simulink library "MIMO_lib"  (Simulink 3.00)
libraries: MIMO_lib x68, simulink3 x1

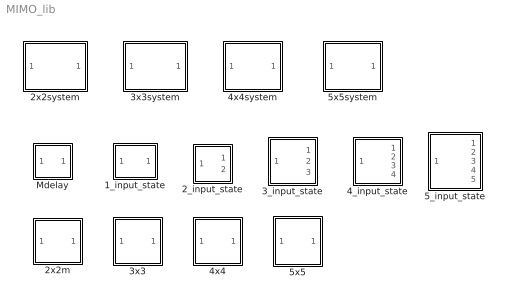
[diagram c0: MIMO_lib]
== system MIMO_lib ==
  1_input_state : Subsystem  mask(SISO_MSF){Ds=}
      mask prompts: Ds "D(s) :"
      mask help: The SISO_MSF block produce, from the input u, a state vector of signal [ ... x''', x'' , x' , x ] to be used further by the K(s) block.
  2_input_state : Subsystem  mask(2_input_state){Ds=}
      mask prompts: Ds "D(s) :"
      mask help: The block generate the state vectors of signal [ ..., x''', x'', x' , x ] of each 2 input signals.
  2x2m : Subsystem  mask(diagonal transferfunction matrix){num=, den=}
      mask prompts: num "diagonal cell array of numurator polynomial"; den "diagonal cell array of denominator polynomial"
      mask help: A block for the simulation of diagonal transfer function matrix, for example the prefilter, and qd part of the feed back controller.
  2x2system : Subsystem  mask(2x2 system){num=, den=, dead=}
      mask prompts: num "numerator :"; den "denominator:"; dead "dead time:"
      mask help: The system is described by a cell array of numerator polynomial, a cell array denominator polynomial of s , and a cell array of dead time.
  3_input_state : Subsystem  mask(3_input_state){Ds=}
      mask prompts: Ds "D(s) :"
      mask help: The block generate the state vectors of signal [ ..., x''', x'', x' , x ] of each 3 input signals.
  3x3 : Subsystem  mask(diagonal transfer function matrix){num=, den=}
      mask prompts: num "diagonal cell array of numurator polynomial"; den "diagonal cell array of denominator polynomial"
      mask help: A block for the simulation of diagonal transfer function matrix, for example the prefilter, and qd part of the feed back controller.
  3x3system : Subsystem  mask(3x3 system){num=, den=, dead=}
      mask prompts: num "numerator"; den "denominator :"; dead "dead time :"
      mask help: The system is described by a cell array of numerator polynomial, a cell array denominator polynomial of s , and a cell array of dead time.
  4_input_state : Subsystem  mask(4_input_state){Ds=}
      mask prompts: Ds "D(s) :"
      mask help: The block generate the state vectors of signal [ ..., x''', x'', x' , x ] of each 4 input signals.
  4x4 : Subsystem  mask(diagonal transfer function matrix){num=, den=}
      mask prompts: num "diagonal cell array of numurator polynomial"; den "diagonal cell array of denominator polynomial"
      mask help: A block for the simulation of diagonal transfer function matrix, for example the prefilter, and qd part of the feed back controller.
  4x4system : Subsystem  mask(4x4 system){num=, den=, dead=}
      mask prompts: num "numerator :"; den "denominator :"; dead "dead time :"
      mask help: The system is described by a cell array of numerator polynomial, a cell array denominator polynomial of s , and a cell array of dead time.
  5_input_state : Subsystem  mask(5_input_state){Ds=}
      mask prompts: Ds "D(s) :"
      mask help: The block generate the state vectors of signal [ ..., x''', x'', x' , x ] of each 5 input signals.
  5x5 : Subsystem  mask(diagonal transfer function matrix){num=, den=}
      mask prompts: num "diagonal cell array of numurator polynomial"; den "diagonal cell array of denominator polynomial"
      mask help: A block for the simulation of diagonal transfer function matrix, for example the prefilter, and qd part of the feed back controller.
  5x5system : Subsystem  mask(5x5 system){num=, den=, dead=}
      mask prompts: num "numerator :"; den "denominator :"; dead "dead time :"
      mask help: The system is described by a cell array of numerator polynomial, a cell array denominator polynomial of s , and a cell array of dead time.
  Mdelay : Subsystem  mask(Mdelay){Mdelay=}
      mask prompts: Mdelay "Delay time:"
      mask help: The modified transport delay that directly feed the signal through when delay time = 0 (to avoid warning if the original Transport delay block is used)

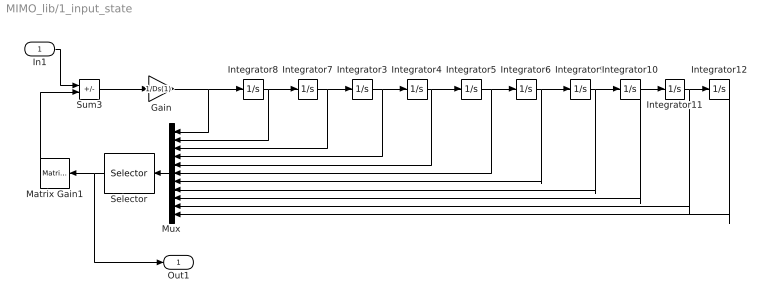
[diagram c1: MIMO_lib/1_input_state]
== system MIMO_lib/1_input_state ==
  In1 : Inport  Port=1  PortWidth=-1  SampleTime=-1  DataType=auto
  Gain : Gain  Gain=1/Ds(1)  SaturateOnIntegerOverflow=on
  Integrator{3..12} (10 alike) : Integrator  ExternalReset=none  InitialConditionSource=internal  InitialCondition=0  LimitOutput=off  UpperSaturationLimit=inf  LowerSaturationLimit=-inf  ShowSaturationPort=off  ShowStatePort=off  AbsoluteTolerance=auto
  Matrix Gain1 : simulink3/Math/Matrix Gain  Orientation=left  K=[0 Ds(2:end)]
  Mux : Mux  Orientation=left  Inputs=11
  Selector : Selector  Orientation=left  Elements=[1 :length(Ds)]  InputPortWidth=11
  Sum3 : Sum  Inputs=+-  SaturateOnIntegerOverflow=on
  Out1 : Outport  Port=1
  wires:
  Sum3/1 -> Gain/1
  In1/1 -> Sum3/1
  Matrix Gain1/1 -> Sum3/2
  Gain/1 -> Integrator8/1, Mux/1
  Integrator8/1 -> Integrator7/1, Mux/2
  Integrator7/1 -> Integrator3/1, Mux/3
  Integrator3/1 -> Integrator4/1, Mux/4
  Integrator4/1 -> Integrator5/1, Mux/5
  Integrator5/1 -> Integrator6/1, Mux/6
  Integrator6/1 -> Integrator9/1, Mux/7
  Integrator9/1 -> Integrator10/1, Mux/8
  Integrator10/1 -> Integrator11/1, Mux/9
  Integrator11/1 -> Integrator12/1, Mux/10
  Integrator12/1 -> Mux/11
  Mux/1 -> Selector/1
  Selector/1 -> Matrix Gain1/1, Out1/1

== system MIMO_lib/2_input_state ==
  In1 : Inport  Port=1  PortWidth=-1  SampleTime=-1  DataType=auto
  1_input_state : MIMO_lib/1_input_state  Ds=Ds{1}
  1_input_state1 : MIMO_lib/1_input_state  Ds=Ds{2}
  Demux : Demux  Outputs=2
  Out1 : Outport  Port=1
  Out2 : Outport  Port=2
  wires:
  Demux/1 -> 1_input_state/1
  Demux/2 -> 1_input_state1/1
  1_input_state/1 -> Out1/1
  In1/1 -> Demux/1
  1_input_state1/1 -> Out2/1

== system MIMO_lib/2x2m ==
  In1 : Inport  Port=1  PortWidth=-1  SampleTime=-1  DataType=auto
  Demux : Demux  Outputs=2
  Mux : Mux  Inputs=2
  Transfer Fcn : TransferFcn  Numerator=num{1,1}  Denominator=den{1,1}
  Transfer Fcn1 : TransferFcn  Numerator=num{2,2}  Denominator=den{2,2}
  Out1 : Outport  Port=1
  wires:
  Demux/1 -> Transfer Fcn/1
  Demux/2 -> Transfer Fcn1/1
  Transfer Fcn/1 -> Mux/1
  Transfer Fcn1/1 -> Mux/2
  Mux/1 -> Out1/1
  In1/1 -> Demux/1

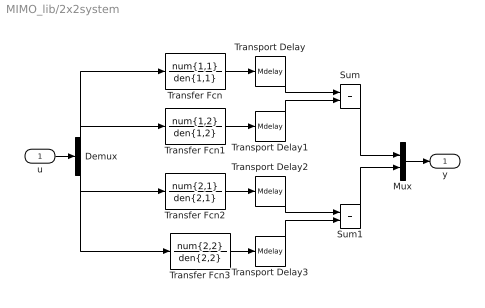
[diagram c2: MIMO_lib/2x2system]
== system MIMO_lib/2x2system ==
  u : Inport  Port=1  PortWidth=-1  SampleTime=-1  DataType=auto
  Demux : Demux  Outputs=2
  Mux : Mux  Inputs=2
  Sum : Sum  Inputs=|++  SaturateOnIntegerOverflow=on
  Sum1 : Sum  Inputs=|++  SaturateOnIntegerOverflow=on
  Transfer Fcn : TransferFcn  Numerator=num{1,1}  Denominator=den{1,1}
  Transfer Fcn1 : TransferFcn  Numerator=num{1,2}  Denominator=den{1,2}
  Transfer Fcn2 : TransferFcn  Numerator=num{2,1}  Denominator=den{2,1}
  Transfer Fcn3 : TransferFcn  Numerator=num{2,2}  Denominator=den{2,2}
  Transport Delay : MIMO_lib/Mdelay  Mdelay=dead{1,1}
  Transport Delay1 : MIMO_lib/Mdelay  Mdelay=dead{1,2}
  Transport Delay2 : MIMO_lib/Mdelay  Mdelay=dead{2,1}
  Transport Delay3 : MIMO_lib/Mdelay  Mdelay=dead{2,2}
  y : Outport  Port=1
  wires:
  Transfer Fcn/1 -> Transport Delay/1
  Transfer Fcn1/1 -> Transport Delay1/1
  Transport Delay/1 -> Sum/1
  Transport Delay1/1 -> Sum/2
  Demux/1 -> Transfer Fcn/1, Transfer Fcn2/1
  Demux/2 -> Transfer Fcn1/1, Transfer Fcn3/1
  Transfer Fcn2/1 -> Transport Delay2/1
  Transfer Fcn3/1 -> Transport Delay3/1
  Transport Delay2/1 -> Sum1/1
  Transport Delay3/1 -> Sum1/2
  Sum/1 -> Mux/1
  Sum1/1 -> Mux/2
  u/1 -> Demux/1
  Mux/1 -> y/1

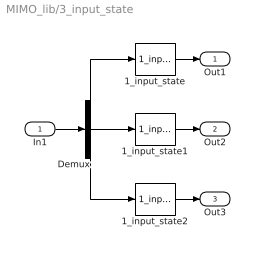
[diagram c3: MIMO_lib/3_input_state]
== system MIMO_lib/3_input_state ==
  In1 : Inport  Port=1  PortWidth=-1  SampleTime=-1  DataType=auto
  1_input_state : MIMO_lib/1_input_state  Ds=Ds{1}
  1_input_state1 : MIMO_lib/1_input_state  Ds=Ds{2}
  1_input_state2 : MIMO_lib/1_input_state  Ds=Ds{3}
  Demux : Demux  Outputs=3
  Out1 : Outport  Port=1
  Out2 : Outport  Port=2
  Out3 : Outport  Port=3
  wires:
  Demux/1 -> 1_input_state/1
  Demux/2 -> 1_input_state1/1
  1_input_state/1 -> Out1/1
  In1/1 -> Demux/1
  1_input_state1/1 -> Out2/1
  1_input_state2/1 -> Out3/1
  Demux/3 -> 1_input_state2/1

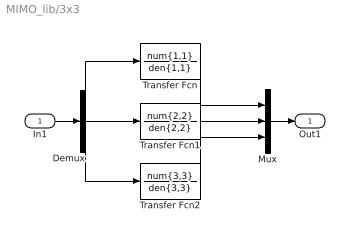
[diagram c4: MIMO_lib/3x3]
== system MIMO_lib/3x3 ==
  In1 : Inport  Port=1  PortWidth=-1  SampleTime=-1  DataType=auto
  Demux : Demux  Outputs=3
  Mux : Mux  Inputs=3
  Transfer Fcn : TransferFcn  Numerator=num{1,1}  Denominator=den{1,1}
  Transfer Fcn1 : TransferFcn  Numerator=num{2,2}  Denominator=den{2,2}
  Transfer Fcn2 : TransferFcn  Numerator=num{3,3}  Denominator=den{3,3}
  Out1 : Outport  Port=1
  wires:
  Transfer Fcn/1 -> Mux/1
  Transfer Fcn1/1 -> Mux/2
  Transfer Fcn2/1 -> Mux/3
  Demux/2 -> Transfer Fcn1/1
  Demux/1 -> Transfer Fcn/1
  Demux/3 -> Transfer Fcn2/1
  Mux/1 -> Out1/1
  In1/1 -> Demux/1

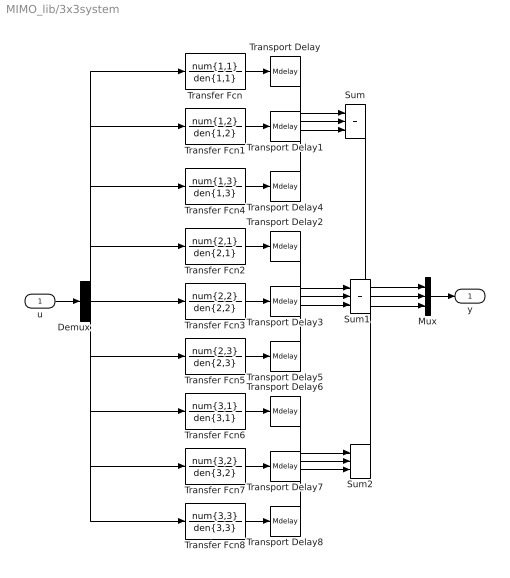
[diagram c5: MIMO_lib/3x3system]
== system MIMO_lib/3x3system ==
  u : Inport  Port=1  PortWidth=-1  SampleTime=-1  DataType=auto
  Demux : Demux  Outputs=3
  Mux : Mux  Inputs=3
  Sum : Sum  Inputs=|+++  SaturateOnIntegerOverflow=on
  Sum1 : Sum  Inputs=|+++  SaturateOnIntegerOverflow=on
  Sum2 : Sum  Inputs=|+++  SaturateOnIntegerOverflow=on
  Transfer Fcn : TransferFcn  Numerator=num{1,1}  Denominator=den{1,1}
  Transfer Fcn1 : TransferFcn  Numerator=num{1,2}  Denominator=den{1,2}
  Transfer Fcn2 : TransferFcn  Numerator=num{2,1}  Denominator=den{2,1}
  Transfer Fcn3 : TransferFcn  Numerator=num{2,2}  Denominator=den{2,2}
  Transfer Fcn4 : TransferFcn  Numerator=num{1,3}  Denominator=den{1,3}
  Transfer Fcn5 : TransferFcn  Numerator=num{2,3}  Denominator=den{2,3}
  Transfer Fcn6 : TransferFcn  Numerator=num{3,1}  Denominator=den{3,1}
  Transfer Fcn7 : TransferFcn  Numerator=num{3,2}  Denominator=den{3,2}
  Transfer Fcn8 : TransferFcn  Numerator=num{3,3}  Denominator=den{3,3}
  Transport Delay : MIMO_lib/Mdelay  Mdelay=dead{1,1}
  Transport Delay1 : MIMO_lib/Mdelay  Mdelay=dead{1,2}
  Transport Delay2 : MIMO_lib/Mdelay  Mdelay=dead{2,1}
  Transport Delay3 : MIMO_lib/Mdelay  Mdelay=dead{2,2}
  Transport Delay4 : MIMO_lib/Mdelay  Mdelay=dead{1,3}
  Transport Delay5 : MIMO_lib/Mdelay  Mdelay=dead{2,3}
  Transport Delay6 : MIMO_lib/Mdelay  Mdelay=dead{3,1}
  Transport Delay7 : MIMO_lib/Mdelay  Mdelay=dead{3,2}
  Transport Delay8 : MIMO_lib/Mdelay  Mdelay=dead{3,3}
  y : Outport  Port=1
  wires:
  Transfer Fcn/1 -> Transport Delay/1
  Transfer Fcn1/1 -> Transport Delay1/1
  Sum/1 -> Mux/1
  Sum1/1 -> Mux/2
  Transfer Fcn2/1 -> Transport Delay2/1
  Transport Delay/1 -> Sum/1
  Transport Delay1/1 -> Sum/2
  Transfer Fcn4/1 -> Transport Delay4/1
  Transfer Fcn3/1 -> Transport Delay3/1
  Transfer Fcn5/1 -> Transport Delay5/1
  Transport Delay2/1 -> Sum1/1
  Demux/1 -> Transfer Fcn/1, Transfer Fcn2/1, Transfer Fcn6/1
  Demux/2 -> Transfer Fcn1/1, Transfer Fcn3/1, Transfer Fcn7/1
  Demux/3 -> Transfer Fcn4/1, Transfer Fcn5/1, Transfer Fcn8/1
  Transport Delay3/1 -> Sum1/2
  Transport Delay5/1 -> Sum1/3
  Transfer Fcn6/1 -> Transport Delay6/1
  Transfer Fcn7/1 -> Transport Delay7/1
  Transfer Fcn8/1 -> Transport Delay8/1
  Transport Delay6/1 -> Sum2/1
  Transport Delay7/1 -> Sum2/2
  Transport Delay8/1 -> Sum2/3
  Sum2/1 -> Mux/3
  Mux/1 -> y/1
  u/1 -> Demux/1
  Transport Delay4/1 -> Sum/3

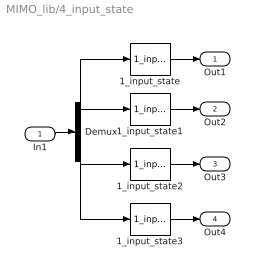
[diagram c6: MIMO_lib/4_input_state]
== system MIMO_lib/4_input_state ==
  In1 : Inport  Port=1  PortWidth=-1  SampleTime=-1  DataType=auto
  1_input_state : MIMO_lib/1_input_state  Ds=Ds{1}
  1_input_state1 : MIMO_lib/1_input_state  Ds=Ds{2}
  1_input_state2 : MIMO_lib/1_input_state  Ds=Ds{3}
  1_input_state3 : MIMO_lib/1_input_state  Ds=Ds{4}
  Demux : Demux  Outputs=4
  Out1 : Outport  Port=1
  Out2 : Outport  Port=2
  Out3 : Outport  Port=3
  Out4 : Outport  Port=4
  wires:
  Demux/1 -> 1_input_state/1
  1_input_state/1 -> Out1/1
  In1/1 -> Demux/1
  1_input_state1/1 -> Out2/1
  1_input_state2/1 -> Out3/1
  Demux/3 -> 1_input_state2/1
  1_input_state3/1 -> Out4/1
  Demux/2 -> 1_input_state1/1
  Demux/4 -> 1_input_state3/1

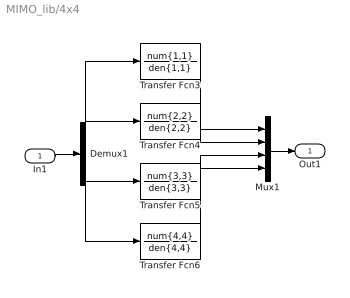
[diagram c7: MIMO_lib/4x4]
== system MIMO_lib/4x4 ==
  In1 : Inport  Port=1  PortWidth=-1  SampleTime=-1  DataType=auto
  Demux1 : Demux  Outputs=4
  Mux1 : Mux  Inputs=4
  Transfer Fcn3 : TransferFcn  Numerator=num{1,1}  Denominator=den{1,1}
  Transfer Fcn4 : TransferFcn  Numerator=num{2,2}  Denominator=den{2,2}
  Transfer Fcn5 : TransferFcn  Numerator=num{3,3}  Denominator=den{3,3}
  Transfer Fcn6 : TransferFcn  Numerator=num{4,4}  Denominator=den{4,4}
  Out1 : Outport  Port=1
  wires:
  Transfer Fcn3/1 -> Mux1/1
  Transfer Fcn5/1 -> Mux1/3
  Demux1/1 -> Transfer Fcn3/1
  Demux1/3 -> Transfer Fcn5/1
  Demux1/4 -> Transfer Fcn6/1
  Transfer Fcn4/1 -> Mux1/2
  Demux1/2 -> Transfer Fcn4/1
  Transfer Fcn6/1 -> Mux1/4
  Mux1/1 -> Out1/1
  In1/1 -> Demux1/1

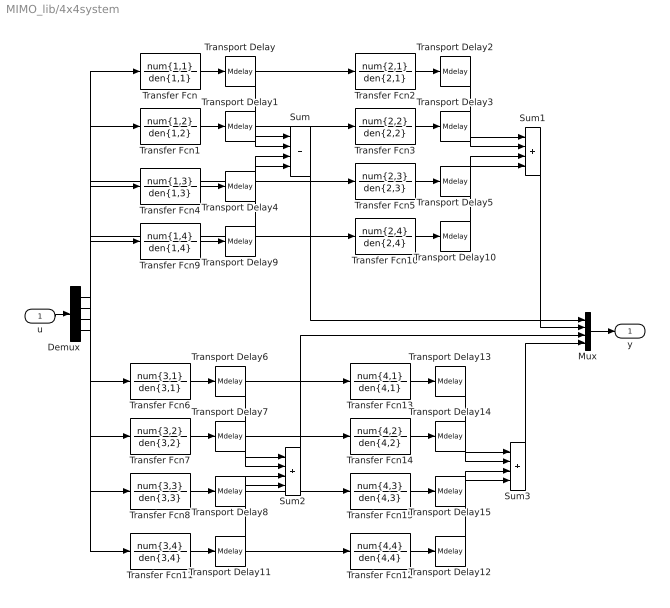
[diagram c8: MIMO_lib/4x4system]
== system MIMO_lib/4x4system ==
  u : Inport  Port=1  PortWidth=-1  SampleTime=-1  DataType=auto
  Demux : Demux  Outputs=4
  Mux : Mux  Inputs=4
  Sum{,1..3} (4 alike) : Sum  Inputs=|++++  SaturateOnIntegerOverflow=on
  Transfer Fcn : TransferFcn  Numerator=num{1,1}  Denominator=den{1,1}
  Transfer Fcn1 : TransferFcn  Numerator=num{1,2}  Denominator=den{1,2}
  Transfer Fcn10 : TransferFcn  Numerator=num{2,4}  Denominator=den{2,4}
  Transfer Fcn11 : TransferFcn  Numerator=num{3,4}  Denominator=den{3,4}
  Transfer Fcn12 : TransferFcn  Numerator=num{4,4}  Denominator=den{4,4}
  Transfer Fcn13 : TransferFcn  Numerator=num{4,1}  Denominator=den{4,1}
  Transfer Fcn14 : TransferFcn  Numerator=num{4,2}  Denominator=den{4,2}
  Transfer Fcn15 : TransferFcn  Numerator=num{4,3}  Denominator=den{4,3}
  Transfer Fcn2 : TransferFcn  Numerator=num{2,1}  Denominator=den{2,1}
  Transfer Fcn3 : TransferFcn  Numerator=num{2,2}  Denominator=den{2,2}
  Transfer Fcn4 : TransferFcn  Numerator=num{1,3}  Denominator=den{1,3}
  Transfer Fcn5 : TransferFcn  Numerator=num{2,3}  Denominator=den{2,3}
  Transfer Fcn6 : TransferFcn  Numerator=num{3,1}  Denominator=den{3,1}
  Transfer Fcn7 : TransferFcn  Numerator=num{3,2}  Denominator=den{3,2}
  Transfer Fcn8 : TransferFcn  Numerator=num{3,3}  Denominator=den{3,3}
  Transfer Fcn9 : TransferFcn  Numerator=num{1,4}  Denominator=den{1,4}
  Transport Delay : MIMO_lib/Mdelay  Mdelay=dead{1,1}
  Transport Delay1 : MIMO_lib/Mdelay  Mdelay=dead{1,2}
  Transport Delay10 : MIMO_lib/Mdelay  Mdelay=dead{2,4}
  Transport Delay11 : MIMO_lib/Mdelay  Mdelay=dead{3,4}
  Transport Delay12 : MIMO_lib/Mdelay  Mdelay=dead{4,4}
  Transport Delay13 : MIMO_lib/Mdelay  Mdelay=dead{4,1}
  Transport Delay14 : MIMO_lib/Mdelay  Mdelay=dead{4,2}
  Transport Delay15 : MIMO_lib/Mdelay  Mdelay=dead{4,3}
  Transport Delay2 : MIMO_lib/Mdelay  Mdelay=dead{2,1}
  Transport Delay3 : MIMO_lib/Mdelay  Mdelay=dead{2,2}
  Transport Delay4 : MIMO_lib/Mdelay  Mdelay=dead{1,3}
  Transport Delay5 : MIMO_lib/Mdelay  Mdelay=dead{2,3}
  Transport Delay6 : MIMO_lib/Mdelay  Mdelay=dead{3,1}
  Transport Delay7 : MIMO_lib/Mdelay  Mdelay=dead{3,2}
  Transport Delay8 : MIMO_lib/Mdelay  Mdelay=dead{3,3}
  Transport Delay9 : MIMO_lib/Mdelay  Mdelay=dead{1,4}
  y : Outport  Port=1
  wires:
  Transfer Fcn/1 -> Transport Delay/1
  Transfer Fcn1/1 -> Transport Delay1/1
  Transfer Fcn4/1 -> Transport Delay4/1
  Transfer Fcn9/1 -> Transport Delay9/1
  u/1 -> Demux/1
  Transfer Fcn2/1 -> Transport Delay2/1
  Transfer Fcn3/1 -> Transport Delay3/1
  Transfer Fcn5/1 -> Transport Delay5/1
  Transfer Fcn10/1 -> Transport Delay10/1
  Transfer Fcn6/1 -> Transport Delay6/1
  Transfer Fcn7/1 -> Transport Delay7/1
  Transfer Fcn8/1 -> Transport Delay8/1
  Transfer Fcn11/1 -> Transport Delay11/1
  Transfer Fcn13/1 -> Transport Delay13/1
  Transfer Fcn14/1 -> Transport Delay14/1
  Transfer Fcn15/1 -> Transport Delay15/1
  Transfer Fcn12/1 -> Transport Delay12/1
  Mux/1 -> y/1
  Transport Delay/1 -> Sum/1
  Transport Delay1/1 -> Sum/2
  Transport Delay4/1 -> Sum/3
  Transport Delay9/1 -> Sum/4
  Sum/1 -> Mux/1
  Transport Delay2/1 -> Sum1/1
  Transport Delay3/1 -> Sum1/2
  Transport Delay5/1 -> Sum1/3
  Transport Delay10/1 -> Sum1/4
  Demux/3 -> Transfer Fcn4/1, Transfer Fcn5/1, Transfer Fcn8/1, Transfer Fcn15/1
  Demux/4 -> Transfer Fcn9/1, Transfer Fcn10/1, Transfer Fcn11/1, Transfer Fcn12/1
  Sum1/1 -> Mux/2
  Transport Delay6/1 -> Sum2/1
  Transport Delay7/1 -> Sum2/2
  Transport Delay8/1 -> Sum2/3
  Transport Delay11/1 -> Sum2/4
  Sum2/1 -> Mux/3
  Sum3/1 -> Mux/4
  Transport Delay13/1 -> Sum3/1
  Transport Delay14/1 -> Sum3/2
  Transport Delay15/1 -> Sum3/3
  Transport Delay12/1 -> Sum3/4
  Demux/2 -> Transfer Fcn1/1, Transfer Fcn3/1, Transfer Fcn7/1, Transfer Fcn14/1
  Demux/1 -> Transfer Fcn/1, Transfer Fcn2/1, Transfer Fcn6/1, Transfer Fcn13/1

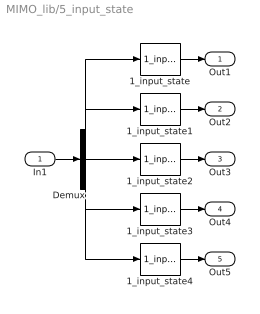
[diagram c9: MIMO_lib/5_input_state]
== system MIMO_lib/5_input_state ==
  In1 : Inport  Port=1  PortWidth=-1  SampleTime=-1  DataType=auto
  1_input_state : MIMO_lib/1_input_state  Ds=Ds{1}
  1_input_state1 : MIMO_lib/1_input_state  Ds=Ds{2}
  1_input_state2 : MIMO_lib/1_input_state  Ds=Ds{3}
  1_input_state3 : MIMO_lib/1_input_state  Ds=Ds{4}
  1_input_state4 : MIMO_lib/1_input_state  Ds=Ds{5}
  Demux : Demux  Outputs=5
  Out1 : Outport  Port=1
  Out2 : Outport  Port=2
  Out3 : Outport  Port=3
  Out4 : Outport  Port=4
  Out5 : Outport  Port=5
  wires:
  Demux/1 -> 1_input_state/1
  1_input_state/1 -> Out1/1
  In1/1 -> Demux/1
  1_input_state1/1 -> Out2/1
  1_input_state2/1 -> Out3/1
  Demux/3 -> 1_input_state2/1
  1_input_state3/1 -> Out4/1
  Demux/2 -> 1_input_state1/1
  Demux/4 -> 1_input_state3/1
  1_input_state4/1 -> Out5/1
  Demux/5 -> 1_input_state4/1

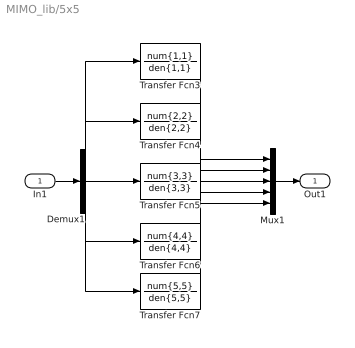
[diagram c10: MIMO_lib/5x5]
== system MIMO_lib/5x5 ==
  In1 : Inport  Port=1  PortWidth=-1  SampleTime=-1  DataType=auto
  Demux1 : Demux  Outputs=5
  Mux1 : Mux  Inputs=5
  Transfer Fcn3 : TransferFcn  Numerator=num{1,1}  Denominator=den{1,1}
  Transfer Fcn4 : TransferFcn  Numerator=num{2,2}  Denominator=den{2,2}
  Transfer Fcn5 : TransferFcn  Numerator=num{3,3}  Denominator=den{3,3}
  Transfer Fcn6 : TransferFcn  Numerator=num{4,4}  Denominator=den{4,4}
  Transfer Fcn7 : TransferFcn  Numerator=num{5,5}  Denominator=den{5,5}
  Out1 : Outport  Port=1
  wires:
  Transfer Fcn3/1 -> Mux1/1
  Transfer Fcn5/1 -> Mux1/3
  Demux1/1 -> Transfer Fcn3/1
  Demux1/3 -> Transfer Fcn5/1
  Demux1/4 -> Transfer Fcn6/1
  Transfer Fcn4/1 -> Mux1/2
  Demux1/2 -> Transfer Fcn4/1
  Transfer Fcn6/1 -> Mux1/4
  Demux1/5 -> Transfer Fcn7/1
  Transfer Fcn7/1 -> Mux1/5
  Mux1/1 -> Out1/1
  In1/1 -> Demux1/1

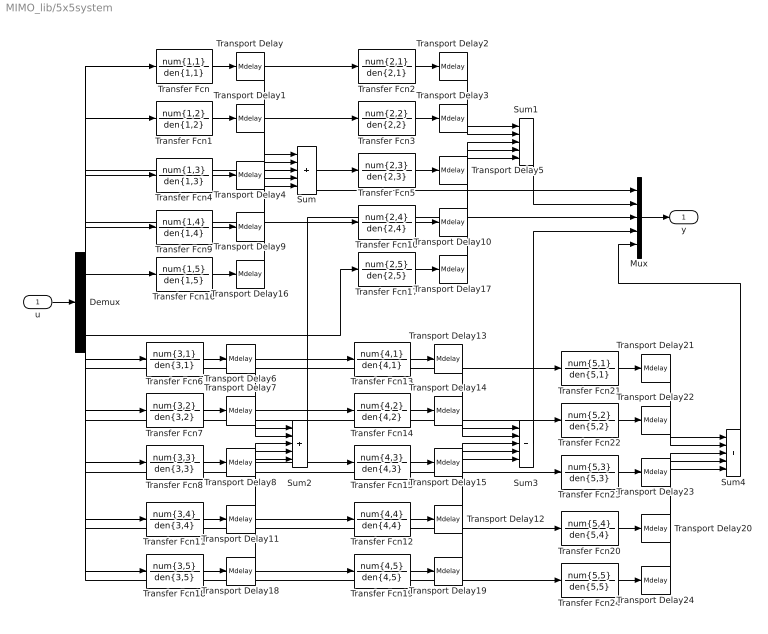
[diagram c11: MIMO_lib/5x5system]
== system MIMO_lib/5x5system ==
  u : Inport  Port=1  PortWidth=-1  SampleTime=-1  DataType=auto
  Demux : Demux  Outputs=5
  Mux : Mux  Inputs=5
  Sum{,1..4} (5 alike) : Sum  Inputs=|+++++  SaturateOnIntegerOverflow=on
  Transfer Fcn : TransferFcn  Numerator=num{1,1}  Denominator=den{1,1}
  Transfer Fcn1 : TransferFcn  Numerator=num{1,2}  Denominator=den{1,2}
  Transfer Fcn10 : TransferFcn  Numerator=num{2,4}  Denominator=den{2,4}
  Transfer Fcn11 : TransferFcn  Numerator=num{3,4}  Denominator=den{3,4}
  Transfer Fcn12 : TransferFcn  Numerator=num{4,4}  Denominator=den{4,4}
  Transfer Fcn13 : TransferFcn  Numerator=num{4,1}  Denominator=den{4,1}
  Transfer Fcn14 : TransferFcn  Numerator=num{4,2}  Denominator=den{4,2}
  Transfer Fcn15 : TransferFcn  Numerator=num{4,3}  Denominator=den{4,3}
  Transfer Fcn16 : TransferFcn  Numerator=num{1,5}  Denominator=den{1,5}
  Transfer Fcn17 : TransferFcn  Numerator=num{2,5}  Denominator=den{2,5}
  Transfer Fcn18 : TransferFcn  Numerator=num{3,5}  Denominator=den{3,5}
  Transfer Fcn19 : TransferFcn  Numerator=num{4,5}  Denominator=den{4,5}
  Transfer Fcn2 : TransferFcn  Numerator=num{2,1}  Denominator=den{2,1}
  Transfer Fcn20 : TransferFcn  Numerator=num{5,4}  Denominator=den{5,4}
  Transfer Fcn21 : TransferFcn  Numerator=num{5,1}  Denominator=den{5,1}
  Transfer Fcn22 : TransferFcn  Numerator=num{5,2}  Denominator=den{5,2}
  Transfer Fcn23 : TransferFcn  Numerator=num{5,3}  Denominator=den{5,3}
  Transfer Fcn24 : TransferFcn  Numerator=num{5,5}  Denominator=den{5,5}
  Transfer Fcn3 : TransferFcn  Numerator=num{2,2}  Denominator=den{2,2}
  Transfer Fcn4 : TransferFcn  Numerator=num{1,3}  Denominator=den{1,3}
  Transfer Fcn5 : TransferFcn  Numerator=num{2,3}  Denominator=den{2,3}
  Transfer Fcn6 : TransferFcn  Numerator=num{3,1}  Denominator=den{3,1}
  Transfer Fcn7 : TransferFcn  Numerator=num{3,2}  Denominator=den{3,2}
  Transfer Fcn8 : TransferFcn  Numerator=num{3,3}  Denominator=den{3,3}
  Transfer Fcn9 : TransferFcn  Numerator=num{1,4}  Denominator=den{1,4}
  Transport Delay : MIMO_lib/Mdelay  Mdelay=dead{1,1}
  Transport Delay1 : MIMO_lib/Mdelay  Mdelay=dead{1,2}
  Transport Delay10 : MIMO_lib/Mdelay  Mdelay=dead{2,4}
  Transport Delay11 : MIMO_lib/Mdelay  Mdelay=dead{3,4}
  Transport Delay12 : MIMO_lib/Mdelay  Mdelay=dead{4,4}
  Transport Delay13 : MIMO_lib/Mdelay  Mdelay=dead{4,1}
  Transport Delay14 : MIMO_lib/Mdelay  Mdelay=dead{4,2}
  Transport Delay15 : MIMO_lib/Mdelay  Mdelay=dead{4,3}
  Transport Delay16 : MIMO_lib/Mdelay  Mdelay=dead{1,5}
  Transport Delay17 : MIMO_lib/Mdelay  Mdelay=dead{2,5}
  Transport Delay18 : MIMO_lib/Mdelay  Mdelay=dead{3,5}
  Transport Delay19 : MIMO_lib/Mdelay  Mdelay=dead{4,5}
  Transport Delay2 : MIMO_lib/Mdelay  Mdelay=dead{2,1}
  Transport Delay20 : MIMO_lib/Mdelay  Mdelay=dead{5,4}
  Transport Delay21 : MIMO_lib/Mdelay  Mdelay=dead{5,1}
  Transport Delay22 : MIMO_lib/Mdelay  Mdelay=dead{5,2}
  Transport Delay23 : MIMO_lib/Mdelay  Mdelay=dead{5,3}
  Transport Delay24 : MIMO_lib/Mdelay  Mdelay=dead{5,5}
  Transport Delay3 : MIMO_lib/Mdelay  Mdelay=dead{2,2}
  Transport Delay4 : MIMO_lib/Mdelay  Mdelay=dead{1,3}
  Transport Delay5 : MIMO_lib/Mdelay  Mdelay=dead{2,3}
  Transport Delay6 : MIMO_lib/Mdelay  Mdelay=dead{3,1}
  Transport Delay7 : MIMO_lib/Mdelay  Mdelay=dead{3,2}
  Transport Delay8 : MIMO_lib/Mdelay  Mdelay=dead{3,3}
  Transport Delay9 : MIMO_lib/Mdelay  Mdelay=dead{1,4}
  y : Outport  Port=1
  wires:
  Transfer Fcn/1 -> Transport Delay/1
  Transfer Fcn1/1 -> Transport Delay1/1
  Transfer Fcn4/1 -> Transport Delay4/1
  Transfer Fcn9/1 -> Transport Delay9/1
  u/1 -> Demux/1
  Transfer Fcn2/1 -> Transport Delay2/1
  Transfer Fcn3/1 -> Transport Delay3/1
  Transfer Fcn5/1 -> Transport Delay5/1
  Transfer Fcn10/1 -> Transport Delay10/1
  Transfer Fcn6/1 -> Transport Delay6/1
  Transfer Fcn7/1 -> Transport Delay7/1
  Transfer Fcn8/1 -> Transport Delay8/1
  Transfer Fcn11/1 -> Transport Delay11/1
  Transfer Fcn13/1 -> Transport Delay13/1
  Transfer Fcn14/1 -> Transport Delay14/1
  Transfer Fcn15/1 -> Transport Delay15/1
  Transfer Fcn12/1 -> Transport Delay12/1
  Transfer Fcn16/1 -> Transport Delay16/1
  Transfer Fcn17/1 -> Transport Delay17/1
  Transfer Fcn18/1 -> Transport Delay18/1
  Transfer Fcn19/1 -> Transport Delay19/1
  Transfer Fcn21/1 -> Transport Delay21/1
  Transfer Fcn22/1 -> Transport Delay22/1
  Transfer Fcn23/1 -> Transport Delay23/1
  Transfer Fcn20/1 -> Transport Delay20/1
  Transfer Fcn24/1 -> Transport Delay24/1
  Mux/1 -> y/1
  Transport Delay/1 -> Sum/1
  Transport Delay1/1 -> Sum/2
  Transport Delay4/1 -> Sum/3
  Transport Delay9/1 -> Sum/4
  Transport Delay16/1 -> Sum/5
  Sum/1 -> Mux/1
  Demux/1 -> Transfer Fcn/1, Transfer Fcn2/1, Transfer Fcn6/1, Transfer Fcn13/1, Transfer Fcn21/1
  Demux/2 -> Transfer Fcn1/1, Transfer Fcn3/1, Transfer Fcn7/1, Transfer Fcn14/1, Transfer Fcn22/1
  Demux/3 -> Transfer Fcn4/1, Transfer Fcn5/1, Transfer Fcn8/1, Transfer Fcn15/1, Transfer Fcn23/1
  Demux/4 -> Transfer Fcn9/1, Transfer Fcn10/1, Transfer Fcn11/1, Transfer Fcn12/1, Transfer Fcn20/1
  Demux/5 -> Transfer Fcn16/1, Transfer Fcn17/1, Transfer Fcn18/1, Transfer Fcn19/1, Transfer Fcn24/1
  Transport Delay2/1 -> Sum1/1
  Transport Delay3/1 -> Sum1/2
  Transport Delay5/1 -> Sum1/3
  Transport Delay10/1 -> Sum1/4
  Transport Delay17/1 -> Sum1/5
  Sum1/1 -> Mux/2
  Transport Delay6/1 -> Sum2/1
  Transport Delay7/1 -> Sum2/2
  Transport Delay8/1 -> Sum2/3
  Transport Delay11/1 -> Sum2/4
  Transport Delay18/1 -> Sum2/5
  Sum2/1 -> Mux/3
  Transport Delay13/1 -> Sum3/1
  Transport Delay14/1 -> Sum3/2
  Transport Delay15/1 -> Sum3/3
  Transport Delay12/1 -> Sum3/4
  Transport Delay19/1 -> Sum3/5
  Sum3/1 -> Mux/4
  Transport Delay21/1 -> Sum4/1
  Transport Delay22/1 -> Sum4/2
  Transport Delay23/1 -> Sum4/3
  Transport Delay20/1 -> Sum4/4
  Transport Delay24/1 -> Sum4/5
  Sum4/1 -> Mux/5

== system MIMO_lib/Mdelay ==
  In1 : Inport  Port=1  PortWidth=-1  SampleTime=-1  DataType=auto
  Constant : Constant  Value=Mdelay
  Saturation : Saturate  Orientation=left  UpperLimit=1000  LowerLimit=1e-5
  Switch : Switch  Threshold=1e-5
  Variable Transport Delay : VariableTransportDelay  MaximumDelay=100  InitialInput=0  MaximumPoints=2048
  Out1 : Outport  Port=1
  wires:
  Variable Transport Delay/1 -> Switch/1
  In1/1 -> Variable Transport Delay/1, Switch/3
  Switch/1 -> Out1/1
  Constant/1 -> Switch/2, Saturation/1
  Saturation/1 -> Variable Transport Delay/2
